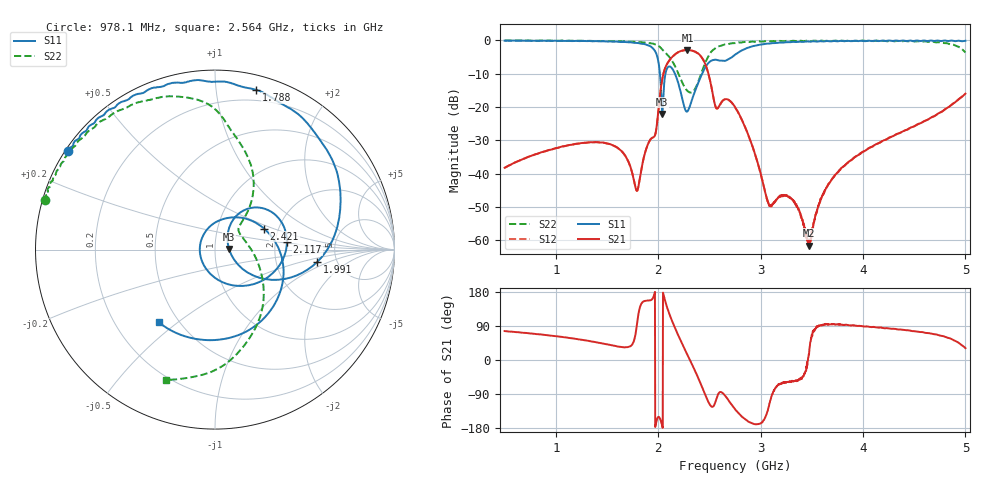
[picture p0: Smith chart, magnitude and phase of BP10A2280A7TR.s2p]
!Agilent Technologies,E8358A,US41080443,A.07.50.56
!Agilent E8358A: A.07.50.56
!Date: Tuesday, December 16, 2014 13:57:36
!Correction: S11(Full 2 Port(1,2))
!S21(Full 2 Port(1,2))
!S12(Full 2 Port(1,2))
!S22(Full 2 Port(1,2))
!S2P File: Measurements: S11, S21, S12, S22:
# Hz S  dB  R 50
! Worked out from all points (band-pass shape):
!   1601 points, 500 MHz to 5 GHz, reference 50 ohm
!   highest |S21| = -2.88 dB at 2.286 GHz (marker M1); lowest = -61.6 dB at 3.476 GHz (marker M2)
!   |S21| within 3 dB of the highest: 2.111 GHz to 2.441 GHz (329.2 MHz wide, 14.5 % of centre)
!   lowest |S11| = -22.1 dB at 2.038 GHz (marker M3), VSWR 1.17, Z = 58.5 + j0.381 ohm
!   |S11| at or under -10 dB: 2.017 GHz to 2.071 GHz (54.28 MHz wide, 2.66 % of centre); 2.164 GHz to 2.429 GHz (265.6 MHz wide, 11.6 % of centre)
!   |S22| runs from -15.7 to 0.0 dB; largest |S21 - S12| = 0.0044
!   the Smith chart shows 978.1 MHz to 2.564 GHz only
!   S11 on the Smith chart (normalised r, x): 978.1 MHz: 0.01, +0.30; 1.788 GHz: 0.11, +1.28; 1.991 GHz: 3.50, -0.74; 2.117 GHz: 2.32, +0.24; 2.421 GHz: 1.68, +0.43; 2.564 GHz: 0.39, -0.43
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5e8  -0.08 163.9  -38.28 76.3  -38.31 76.4  -0.05 172.8
9.78125e8  -0.12 146.3  -32.58 63.8  -32.61 63.9  -0.10 163.8
1.250938e9  -0.18 132.3  -30.85 53.6  -30.91 53.6  -0.13 156.5
1.616562e9  -0.45 101.9  -32.60 35.1  -32.59 35.1  -0.25 140.9
1.788125e9  -0.73 75.6  -45.07 85.2  -45.12 85.0  -0.48 128.5
1.990625e9  -4.86 -7.1  -24.38 -154.7  -24.42 -154.4  -1.43 98.1
2.001875e9  -6.41 -17.5  -21.06 -150.0  -21.05 -149.8  -1.62 95.1
2.038438e9  -22.13 2.4  -11.85 -173.1  -11.92 -173.1  -2.74 86.2
2.117188e9  -7.89 6.3  -5.65 115.6  -5.70 115.8  -5.32 70.0
2.285938e9  -21.32 167.4  -2.88 13.2  -2.92 13.2  -15.23 41.1
2.420938e9  -10.55 23.3  -4.93 -66.8  -4.96 -66.7  -9.91 -33.5
2.564375e9  -5.82 -127.6  -20.23 -105.8  -20.28 -105.7  -2.19 -110.7
2.634688e9  -6.17 153.4  -17.97 -88.6  -17.99 -88.2  -1.36 -131.5
2.75e9  -4.30 43.1  -20.01 -129.8  -20.07 -129.5  -0.83 -152.1
2.854062e9  -2.47 -14.7  -26.39 -157.4  -26.43 -157.7  -0.45 -164.0
3.028438e9  -1.15 -66.2  -43.59 -158.9  -43.54 -159.3  -0.32 -176.2
3.475625e9  -0.39 -119.5  -61.64 23.9  -61.83 30.7  -0.19 165.3
3.500938e9  -0.31 -120.7  -57.48 66.8  -57.37 63.1  -0.18 165.4
3.723125e9  -0.19 -134.2  -40.68 93.9  -40.61 94.2  -0.07 160.3
4.251875e9  -0.04 -154.3  -29.30 83.7  -29.34 83.7  -0.21 149.7
4.74125e9  -0.09 -168.5  -21.88 65.1  -21.90 65.5  -0.55 130.8
5e9  -0.13 -173.2  -16.01 31.2  -16.06 31.2  -3.66 79.5
